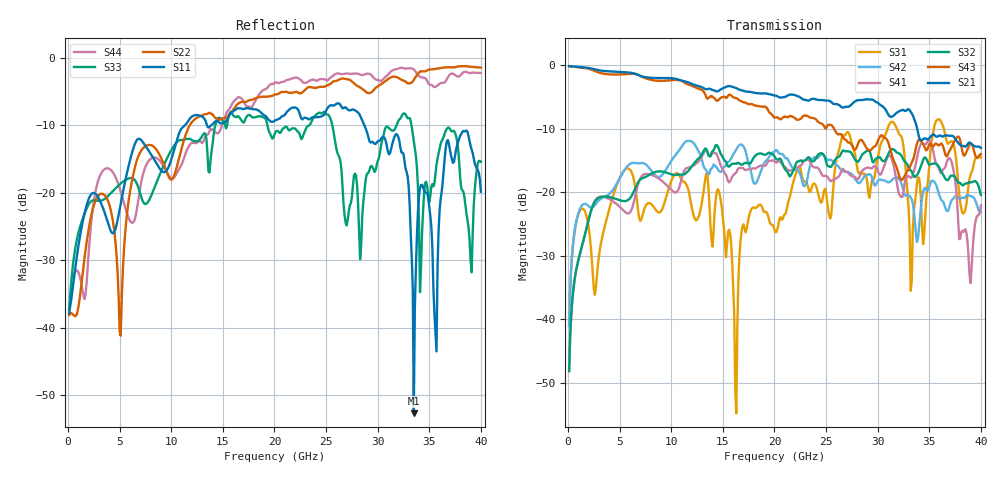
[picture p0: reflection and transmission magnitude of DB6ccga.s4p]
! ADC12DJ3200QML-SP
! 196-pin NWE package
! CCGA Ceramic Package with columns (ceramic column grid array)
! Texas Instruments 4/21/2021
! Single-ended  S-parameters
! PORT#  PORT_NAME  NET_NAME
! PORT1:  DAxN.DIEBUMP DAxN
! PORT2:  DAxN.BGA  DAxN
! PORT3:  DAxP.DIEBUMP DAxP
! PORT4:  DAxP.BGA  DAxP
! Touchstone Ver. 1.0
! Number of ports is 4
# Hz	S	MA	R	50.000000
! SCATTERING PARAMETERS  :
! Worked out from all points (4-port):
!   400 points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, 100 MHz to 40 GHz, reference 50 ohm
!   strongest paths, dB at 100 MHz, 10.1 GHz, 20.1 GHz, 30.1 GHz, 40 GHz:
!     S21: -0.1, -2.0, -4.7, -6.0, -13.0
!     S43: -0.1, -2.3, -8.2, -11.6, -14.0
!     S32: -48.1, -17.2, -14.6, -14.4, -20.4
!     S41: -48.1, -19.7, -15.3, -17.0, -22.0
!     S42: -41.0, -14.8, -13.3, -18.0, -23.1
!     S31: -41.0, -17.8, -26.3, -13.8, -14.5
!   lowest |S11| = -52.6 dB at 33.5 GHz (marker M1), VSWR 1.00, Z = 50.2 + j0.033 ohm
!   |S11| at or under -10 dB: start of sweep to 11.33 GHz; 13.46 GHz to 13.88 GHz (424.6 MHz wide, 3.11 % of centre); 28.7 GHz to end of sweep
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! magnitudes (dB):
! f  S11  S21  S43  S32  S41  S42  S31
! 100 MHz  -37.8  -0.1  -0.1  -48.1  -48.1  -41.0  -41.0
! 13.4 GHz  -9.7  -3.8  -5.0  -13.1  -13.3  -16.5  -17.0
! 16.3 GHz  -7.6  -3.6  -5.1  -15.5  -16.8  -13.3  -54.8
! 26.2 GHz  -6.8  -6.2  -10.8  -14.4  -17.5  -15.9  -13.6
! 32.5 GHz  -14.2  -7.0  -17.7  -14.8  -20.0  -19.7  -12.8
! 33.5 GHz  -52.6  -8.3  -14.5  -17.5  -16.7  -22.8  -23.0
! 40 GHz  -19.9  -13.0  -14.0  -20.4  -22.0  -23.1  -14.5
